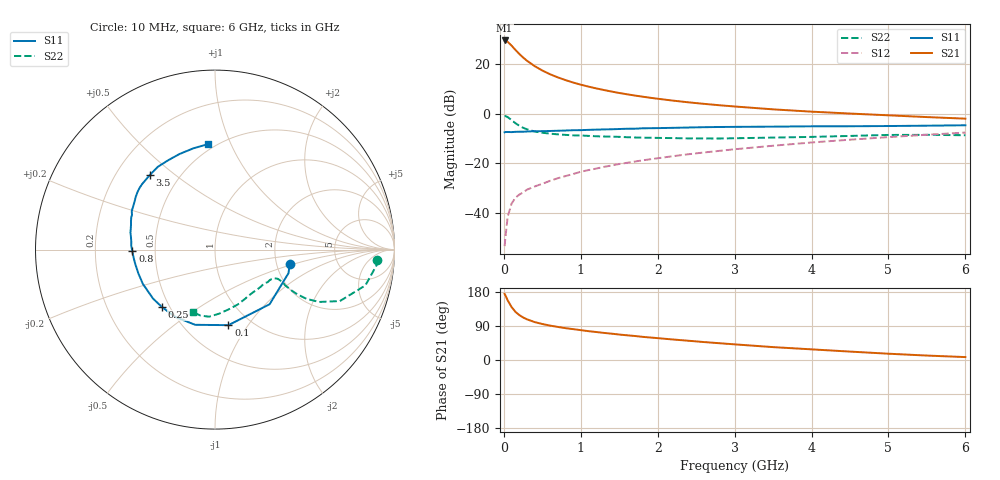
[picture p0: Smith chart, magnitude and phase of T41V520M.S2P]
! Infineon Technologies  Discrete & RF Semiconductors
! BFR182T
! Si NPN RF Bipolar Junction Transistor in SC75
! VCE = 1.5 V  IC = 20 mA
! Common Emitter S-Parameters:  October  1999
# GHz  S  MA  R  50
!  f  S11  S21  S12  S22
! GHz  MAG  ANG  MAG  ANG  MAG  ANG  MAG  ANG
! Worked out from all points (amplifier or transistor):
!   36 points, 10 MHz to 6 GHz, reference 50 ohm
!   highest |S21| = 29.7 dB at 10 MHz (marker M1)
!   |S21| within 3 dB of that: start of sweep to 126.6 MHz
!   unconditionally stable (mu >= 1): start of sweep to 13.46 MHz; 400.8 MHz to 4.518 GHz
!   at 250 MHz: K = 0.80, MSG = 27.3 dB, |S12| = -31.8 dB
!   at 1.4 GHz: K = 1.27, MAG = 11.8 dB, |S12| = -20.9 dB
!   at 6 GHz: K = 0.93, MSG = 2.8 dB, |S12| = -7.6 dB
!   S11 on the Smith chart (normalised r, x): 10 MHz: 2.37, -0.45; 100 MHz: 0.79, -0.82; 250 MHz: 0.46, -0.36; 800 MHz: 0.37, -0.01; 3.5 GHz: 0.34, +0.41; 6 GHz: 0.46, +0.82
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0.01  0.4238 -10.6  30.67 174.4  0.0021 85.6  0.9049 -3.5
0.02  0.4301 -17.7  30.65 170.8  0.0031 80.9  0.9046 -5.5
0.05  0.4305 -45.0  28.76 157.4  0.0083 77.4  0.8612 -13.4
0.1  0.4276 -79.9  24.13 139.9  0.0152 67.1  0.7525 -22.4
0.15  0.4334 -104.8  19.78 127.3  0.02 60.1  0.6492 -26.7
0.2  0.4357 -120.8  16.43 118.7  0.0232 61.9  0.5781 -28.3
0.25  0.4356 -132.7  13.87 112.3  0.0256 59.1  0.5235 -28.5
0.3  0.4401 -141.6  11.94 107.4  0.0292 59.2  0.4887 -28.2
0.4  0.445 -154.5  9.285 100.1  0.0339 60.2  0.4397 -27.0
0.5  0.4471 -162.8  7.562 95.0  0.0385 63.8  0.4154 -25.7
0.6  0.451 -169.4  6.353 90.8  0.0441 65.4  0.3984 -25.2
0.7  0.4558 -174.3  5.496 87.3  0.0498 66.8  0.3856 -25.0
0.8  0.4607 -178.9  4.842 84.1  0.055 68.2  0.3763 -25.3
0.9  0.4671 177.5  4.317 81.5  0.0606 69.4  0.368 -25.7
1.1  0.475 170.8  3.567 76.1  0.0729 69.7  0.3588 -27.3
1.3  0.4847 165.3  3.044 71.5  0.0846 70.6  0.3486 -29.5
1.6  0.5005 158.8  2.495 65.2  0.1022 71.2  0.3374 -33.3
2.2  0.5221 149.1  1.856 54.1  0.1394 70.6  0.3236 -43.5
3.5  0.5521 130.9  1.236 34.0  0.2268 65.6  0.3315 -67.9
4.5  0.5619 117.8  1.016 22.2  0.3004 59.4  0.3579 -86.5
5.5  0.5772 101.9  0.862 11.7  0.3781 52.0  0.3764 -102.3
6  0.5883 94.0  0.801 7.7  0.4189 47.3  0.37 -109.1
